{attribute 'qualified_only'}
VAR_GLOBAL
	HeartBeat:REAL;
//HW
	NDO:STR_NDO;
	AO:STR_AO;
	
//Config
	PMConfig:ConfigPM;
	
	MFCVerification:ConfigMfcVer;
	
	Chiller:ConfigChiller;	
	InnerChiller:ConfigChiller;
	OuterChiller:ConfigChiller;
	TopChiller:ConfigChiller;
	
	DryPump:ConfigDryPump;
	
	Mfcgas1:ConfigMfcGas;
	Mfcgas2:ConfigMfcGas;
	Mfcgas3:ConfigMfcGas;
	Mfcgas4:ConfigMfcGas;
	Mfcgas5:ConfigMfcGas;
	Mfcgas6:ConfigMfcGas;
	Mfcgas7:ConfigMfcGas;
	Mfcgas8:ConfigMfcGas;
	Mfcgas9:ConfigMfcGas;
	Mfcgas10:ConfigMfcGas;
	Mfcgas11:ConfigMfcGas;
	Mfcgas12:ConfigMfcGas;	
	MfcN2:ConfigMfcGas;
	MfcHe:ConfigMfcGas;
	
	Pump:ConfigPump;
	
	Purge:ConfigPurge;
	
	PendulumHeater:ConfigHeater;
	LidHeater:ConfigHeater;
	ChamberHeater:ConfigHeater;
	IGSHeater:ConfigHeater;
	TapeHeater:ConfigHeater;
	ForelineHeater:ConfigHeater;
	STAGE:ConfigHeater;
	
	ElectrostaticVoltageSource:ConfigElectrostaticVoltageSource;
	
	TurboPump:ConfigTurboPump;
	
	PendulumValve:ConfigPendulumValve;
	
	IdleClean:ConfigIdleClean;
	
	EPD:ConfigEPD;
	
	HighTemperatureChiller:ConfigHighTempChiller;
	
	
	
	
//RECIPE
	Step_Num:INT;
	SetpArray:ARRAY[1..100] OF RecipeEachStep;

	
//INTERLOCK
	TurboN2PurgePressure:INT;	//PS103	
	
//PROCESS
	Process_Start:BOOL;
	Process_Stop:BOOL;

//*********************READ**************
//	Process_Finished:BOOL;

//WARNING&ALARM

	Warning_And_Alarm_RST:BOOL;

	
END_VAR
